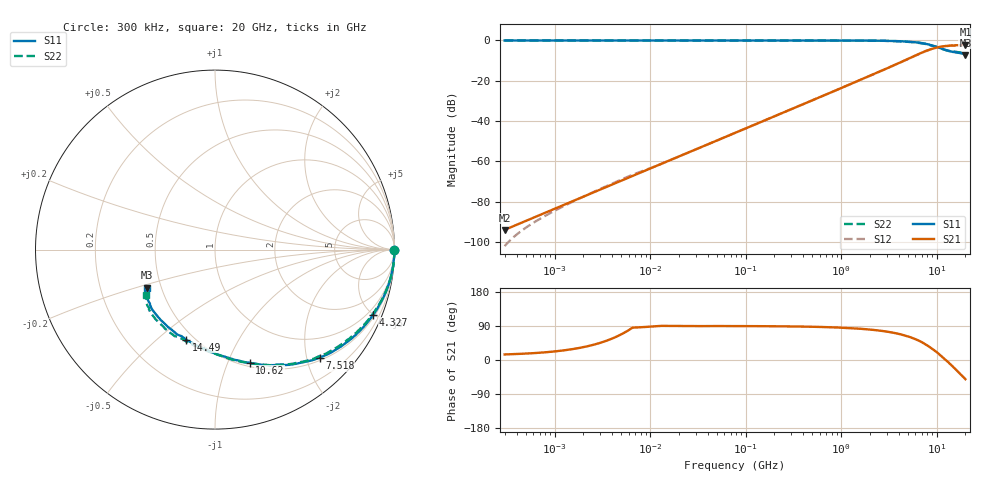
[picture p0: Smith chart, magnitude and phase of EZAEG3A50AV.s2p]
!*** S-Parameter ***
!Copyright (C)  Panasonic Industry
!ESD Suppressor
!Parts No.  EZAEG3A50AV
! Size : 1608mm
# hz S ma R 50
! 2 Port Network Data from SP1.SP block
! freq  magS11  angS11  magS21  angS21  magS12  angS12  magS22  angS22
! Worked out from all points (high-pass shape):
!   966 points, 300 kHz to 20 GHz, reference 50 ohm
!   highest |S21| = -2.04 dB at 20 GHz (marker M1); lowest = -93.9 dB at 300 kHz (marker M2)
!   |S21| within 3 dB of the highest: 7.878 GHz to end of sweep
!   lowest |S11| = -7.2 dB at 20 GHz (marker M3), VSWR 2.55, Z = 20.7 - j10.8 ohm
!   |S11| at or under -10 dB: nowhere
!   |S22| runs from -6.8 to 0.0 dB; largest |S21 - S12| = 0.021
!   S11 on the Smith chart (normalised r, x): 300 kHz: open; 4.327 GHz: 0.62, -4.97; 7.518 GHz: 0.55, -2.24; 10.62 GHz: 0.54, -1.20; 14.49 GHz: 0.45, -0.63; 20 GHz: 0.41, -0.22
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300000  0.9998 0.0  2.009e-05 14.7  7.914e-06 -31.0  1 0.0
1435382  0.9998 0.0  9.613e-05 27.5  9.186e-05 -9.4  1 0.0
1592052  0.9998 0.0  0.0001066 29.3  0.0001034 -6.4  1 0.0
1913988  0.9998 0.0  0.0001282 32.9  0.0001272 -0.3  0.9999 0.0
6336094  0.9998 -0.0  0.0004244 82.9  0.0004542 83.8  1 -0.0
1.221117e7  0.9999 -0.0  0.0008115 89.6  0.0008117 89.5  1 -0.0
7.790674e7  0.9991 -0.3  0.005124 89.5  0.005124 89.5  1 -0.3
4.970419e8  0.9988 -2.2  0.03262 87.7  0.03263 87.6  0.9995 -2.2
1.466516e9  0.995 -6.7  0.0968 83.0  0.09672 82.9  0.9949 -6.9
2.219453e9  0.9887 -10.5  0.1476 79.2  0.1474 79.0  0.9872 -10.7
3.171107e9  0.9763 -15.6  0.2139 74.0  0.213 73.8  0.9727 -15.9
4.326935e9  0.9534 -22.4  0.2973 66.8  0.2959 66.7  0.9472 -22.8
5.83648e9  0.9097 -32.7  0.4118 56.5  0.4074 56.4  0.8999 -33.2
7.518412e9  0.8381 -46.0  0.535 42.4  0.5314 42.9  0.8254 -46.7
8.9353e9  0.7572 -58.1  0.6176 30.0  0.6143 30.2  0.7449 -59.2
1.061921e10  0.659 -73.0  0.6881 15.6  0.6813 15.7  0.6507 -74.9
1.233325e10  0.5843 -88.4  0.7238 0.9  0.7229 1.9  0.5782 -90.5
1.448978e10  0.5261 -107.7  0.75 -15.1  0.7498 -14.4  0.5326 -108.7
1.607132e10  0.5044 -121.3  0.762 -26.4  0.7624 -25.4  0.5215 -122.2
1.741982e10  0.4884 -132.3  0.7636 -35.1  0.7686 -34.0  0.5069 -132.0
1.866538e10  0.4694 -142.3  0.7632 -43.1  0.7725 -42.2  0.4902 -140.1
2e10  0.4362 -151.0  0.7908 -50.7  0.7971 -49.8  0.4584 -146.4
